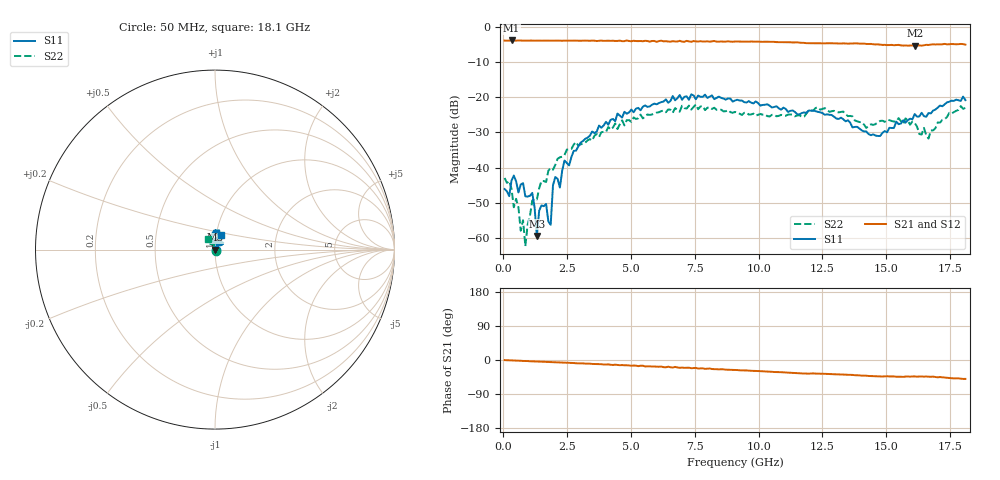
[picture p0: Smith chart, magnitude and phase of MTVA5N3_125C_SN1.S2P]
! Network Analyzer HP8720D.06.14 Serial No. US36140669
! 11 May 2005  11:50:53
! Frequency  S11  S21  S12  S22
# HZ  S  DB R 50
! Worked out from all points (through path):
!   201 points, 50 MHz to 18.1 GHz, reference 50 ohm
!   highest |S21| = -3.92 dB at 320.8 MHz (marker M1); lowest = -5.4 dB at 16.11 GHz (marker M2)
!   group delay of S21, straight-line fit = 7.69 ps
!   lowest |S11| = -59.4 dB at 1.313 GHz (marker M3), VSWR 1.00, Z = 49.9 - j0.0576 ohm
!   |S11| at or under -10 dB: start of sweep to end of sweep
!   |S22| runs from -62.3 to -22.1 dB; largest |S21 - S12| = 0.023
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5e7  -46.08 -51.6  -3.95 -0.3  -3.96 -0.6  -42.95 -64.9
3.2075e8  -43.70 -151.3  -3.92 -1.0  -3.94 -1.3  -46.00 -53.4
5.915e8  -47.07 -143.6  -3.93 -1.7  -3.96 -2.1  -51.29 -30.6
6.8175e8  -44.81 -155.7  -3.95 -2.1  -3.96 -2.5  -57.93 -15.0
7.72e8  -44.42 -139.6  -3.96 -2.5  -3.94 -2.8  -54.92 21.0
8.6225e8  -48.15 -132.6  -3.95 -2.6  -3.97 -3.0  -62.31 104.2
1.133e9  -47.19 -134.6  -3.95 -3.5  -3.97 -3.9  -49.38 79.2
1.3135e9  -59.45 -147.2  -3.96 -4.0  -3.96 -4.2  -49.05 75.5
1.494e9  -50.74 -100.3  -3.98 -4.5  -3.96 -4.9  -43.78 86.2
1.855e9  -56.24 -25.7  -3.98 -5.5  -3.97 -5.8  -40.14 88.9
1.94525e9  -45.02 5.1  -3.99 -5.6  -3.97 -6.2  -40.62 84.5
2.0355e9  -42.68 35.4  -3.98 -6.0  -3.97 -6.4  -39.23 96.1
2.216e9  -45.66 34.6  -3.98 -6.6  -3.95 -6.9  -37.08 84.1
2.3965e9  -38.02 39.3  -3.98 -7.0  -3.97 -7.4  -36.45 91.5
3.1185e9  -32.44 54.0  -3.98 -8.9  -3.99 -9.5  -33.27 112.8
6.09675e9  -21.69 76.3  -4.08 -17.8  -4.03 -18.1  -24.28 77.9
9.075e9  -20.96 95.3  -4.22 -26.4  -4.19 -26.7  -24.22 64.1
1.21435e10  -23.82 101.2  -4.72 -35.4  -4.68 -35.9  -23.80 77.3
1.512175e10  -28.72 50.1  -5.23 -43.4  -5.12 -43.4  -26.54 98.4
1.61145e10  -24.82 39.2  -5.43 -43.3  -5.26 -44.0  -27.37 87.5
1.6656e10  -24.52 52.9  -5.20 -44.1  -5.08 -43.9  -31.77 110.7
1.81e10  -20.85 67.2  -5.11 -49.8  -5.10 -51.3  -23.05 124.0
